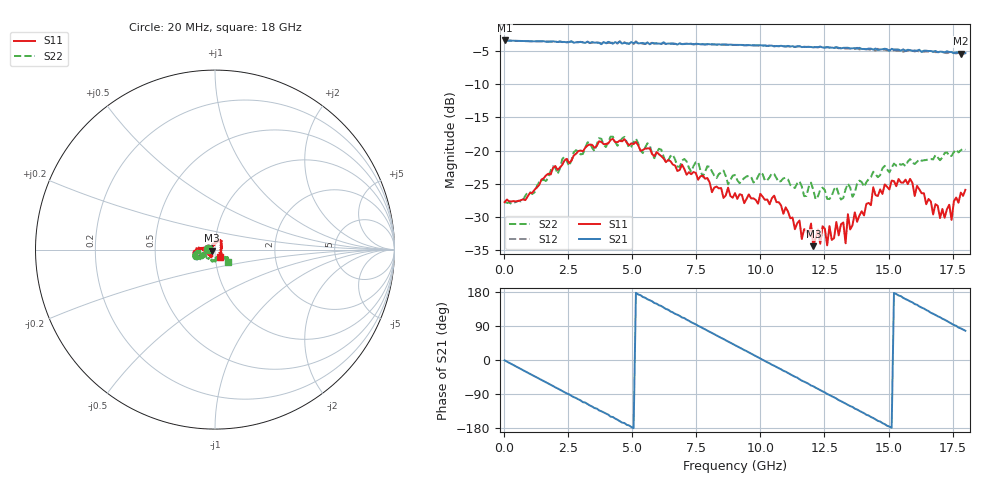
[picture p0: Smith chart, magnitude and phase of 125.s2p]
!Agilent Technologies,N5230A,US43500223,A.07.50.48
!Agilent N5230A: A.07.50.48
!Date: Wednesday, February 17, 2016 15:24:26
!Correction: S11(Full 2 Port(1,2))
!S21(Full 2 Port(1,2))
!S12(Full 2 Port(1,2))
!S22(Full 2 Port(1,2))
!S2P File: Measurements: S11, S21, S12, S22:
# Hz S  RI  R 50
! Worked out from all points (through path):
!   201 points, 20 MHz to 18 GHz, reference 50 ohm
!   highest |S21| = -3.41 dB at 20 MHz (marker M1); lowest = -5.4 dB at 17.82 GHz (marker M2)
!   group delay of S21, straight-line fit = 99.1 ps
!   lowest |S11| = -34.4 dB at 12.07 GHz (marker M3), VSWR 1.04, Z = 48.2 - j0.547 ohm
!   |S11| at or under -10 dB: start of sweep to end of sweep
!   |S22| runs from -28.0 to -17.9 dB; largest |S21 - S12| = 0.032
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2e7  -0.041 0.000853  0.6755 -0.0104  0.6755 -0.0105  -0.041 0.000586
1.5483e9  -0.0561 -0.0264  0.3738 -0.5523  0.3717 -0.5525  -0.05 -0.0334
3.0766e9  -0.0923 -0.0352  -0.237 -0.6077  -0.2344 -0.6125  -0.0868 -0.0374
4.515e9  -0.1167 -0.0245  -0.6269 -0.2108  -0.6337 -0.2101  -0.1135 -0.0246
6.0433e9  -0.0937 0.00439  -0.5217 0.3722  -0.5134 0.3825  -0.1026 -0.0117
7.4817e9  -0.0677 0.00538  -0.0445 0.6366  -0.0318 0.6325  -0.079 -0.0212
9.01e9  -0.0401 -0.0261  0.4836 0.3969  0.4901 0.3867  -0.0424 -0.0498
1.03585e10  -0.0145 -0.0367  0.611 -0.0949  0.6071 -0.1057  -0.0136 -0.0615
1.15272e10  -0.0235 -0.0183  0.3858 -0.4741  0.3782 -0.4808  0.0113 -0.0577
1.16171e10  -0.0197 -0.00895  0.3505 -0.4894  0.3466 -0.4916  0.0181 -0.0505
1.19767e10  -0.0276 -0.006  0.2318 -0.5569  0.2291 -0.5569  0.0141 -0.0557
1.20666e10  -0.0182 -0.00567  0.2118 -0.5602  0.1966 -0.5703  0.0171 -0.0475
1.29656e10  -0.0227 0.0182  -0.1222 -0.5895  -0.1461 -0.5784  0.022 -0.0487
1.33252e10  -0.0111 0.0167  -0.25 -0.5399  -0.2604 -0.526  0.0192 -0.0474
1.34151e10  -0.0155 0.0294  -0.2829 -0.524  -0.2898 -0.511  0.0295 -0.0482
1.3505e10  -0.0135 0.0216  -0.3075 -0.4999  -0.3182 -0.4947  0.0323 -0.0418
1.4404e10  0.0106 0.0519  -0.5137 -0.2609  -0.5222 -0.2427  0.0509 -0.0471
1.50333e10  0.0198 0.047  -0.562 -0.0425  -0.5704 -0.0189  0.0558 -0.0399
1.58424e10  0.0382 0.0479  -0.5164 0.2451  -0.5122 0.2503  0.0718 -0.0481
1.74606e10  0.024 -0.0181  -0.0578 0.5491  -0.0415 0.5477  0.0744 -0.0529
1.78202e10  0.0297 -0.0382  0.0613 0.5351  0.085 0.528  0.0822 -0.0581
1.8e10  0.0284 -0.042  0.1209 0.5291  0.1427 0.5168  0.0744 -0.069
